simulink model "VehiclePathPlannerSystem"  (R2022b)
settings: Solver=VariableStepAuto  StartTime=0.0  StopTime=Tsim  RelTol=1e-3
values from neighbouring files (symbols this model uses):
  distToCenter = 0.5*egoWheelbase    [main.m]
  egoInitialPose = [1, 3, 0]    [main.m]
  egoLength = 4.7    [helperSLVisualizeParking.m]    (also in main.m = vdims.Length; parkingIneqConFcn.m = vdims.Length; parkingIneqConFcnJacobian.m = vdims.Length; parkingStateValidator.m)
  egoTargetPose = [-3.1, -3.15, pi/2]    [main.m]
  egoWheelbase = vdims.Wheelbase    [main.m]
  egoWidth = 1.8    [helperSLVisualizeParking.m]    (also in main.m = vdims.Width; parkingIneqConFcn.m = vdims.Width; parkingIneqConFcnJacobian.m = vdims.Width; parkingStateValidator.m)
  hp = 35    [main.m]    (also in parkingCostFcn.m = data.PredictionHorizon; parkingCostJacobian.m = data.PredictionHorizon; parkingIneqConFcn.m = data.PredictionHorizon; parkingIneqConFcnJacobian.m = data.PredictionHorizon)
  numObs = 8    [main.m]
  obsMat = [-9.3      , -1.75, 0,      egoLength,     egoWidth ;            -obsLength, -1.75, 0,      egoLength,     egoWidth ;             11.35    ,  1.35, 0,  4 * obsLength, 0.5          ;            -1.3      , -2   , 0,  0.5          , 1 + obsLength;            -obsLength, -5.35, 0, 10.3          , 0.5          ;            -11.1     , -2   , 0,  0.5          , 1 + obsLength;            -17.55    ,  1.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    [main.m]
  safetyDistance = 0.1    [main.m]
  steer_range = [-pi/5, pi/5]    [main.m]
  Ts = 0.1    [main.m]
  v_range = [-3.5, 3.5]    [main.m]
undefined symbols (not defined in the file or in its folder): blkObsMat, Column, D, egoParas, numParas, repmat, Row, vector
libraries: mpclib x1

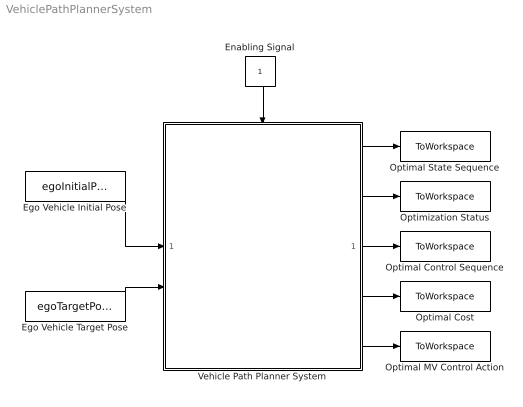
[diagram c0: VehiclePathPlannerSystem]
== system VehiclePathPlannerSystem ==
  Ego Vehicle Initial Pose : Constant  Value=egoInitialPose  VectorParams1D=off
  Ego Vehicle Target Pose : Constant  Value=egoTargetPose  VectorParams1D=off
  Enabling Signal : Constant
  Optimal Control Sequence : ToWorkspace  VariableName=mv_seq  SampleTime=-1
  Optimal Cost : ToWorkspace  VariableName=cost  SampleTime=-1
  Optimal MV Control Action : ToWorkspace  VariableName=mv_opti  SampleTime=-1
  Optimal State Sequence : ToWorkspace  VariableName=x_seq  SampleTime=-1
  Optimization Status : ToWorkspace  VariableName=exitflag  SampleTime=-1
  Vehicle Path Planner System : Subsystem  AncestorBlock=mpclib/Automated Driving/Vehicle Path Planner System  TreatAsAtomicUnit=on  mask(Vehicle Path Planner (VPP) system){egoLength=egoLength, egoWidth=egoWidth, wheelbase=egoWheelbase, dist2Center=distToCenter, numObs=numObs, obsMat=obsMat, obs_ext=off, minDist=safetyDistance, Ts=Ts, pPlanning=hp, v_range=v_range, v_ext=off, steer_range=steer_range, steer_ext=off, suboptimal=off, maxiter=200, output_exitflag=on}
      mask prompts: egoLength "MPC:adasblocks:promptCPPLength"; egoWidth "MPC:adasblocks:promptCPPWidth"; wheelbase "MPC:adasblocks:promptCPPWheelbase"; dist2Center "MPC:adasblocks:promptCPPCenterToRear"; numObs "MPC:adasblocks:promptCPPNumObs"; obsMat "MPC:adasblocks:promptCPPObsList"; obs_ext "MPC:adasblocks:promptCPPUseExternalSource"; minDist "MPC:adasblocks:promptCPPMinDist"; Ts "MPC:adasblocks:promptCPPSampleTime"; pPlanning "MPC:adasblocks:promptCPPSteps"; v_range "MPC:adasblocks:promptCPPVelRange"; v_ext "MPC:adasblocks:promptCPPUseExternalSource"; steer_range "MPC:adasblocks:promptCPPSteerRange"; steer_ext "MPC:adasblocks:promptCPPUseExternalSource"; suboptimal "MPC:adasblocks:promptCPPUseSubOptimal"; maxiter "MPC:adasblocks:promptCPPMaxIter"; output_exitflag "MPC:adasblocks:promptCPPExitflag"
      mask help: MPC:adasblocks:vppMaskDescription
      mask init:
      | [nlobj,numParas,egoParas,blkDataType,blkObsDim,blkObsMat] = vppblock_MaskInitFcn(gcb,pPlanning,Ts,...
      |     wheelbase,egoLength,egoWidth,dist2Center,minDist,...
      |     obsMat,numObs,v_range,steer_range,maxiter);
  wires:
  Enabling Signal/1 -> Vehicle Path Planner System/Enable
  Ego Vehicle Target Pose/1 -> Vehicle Path Planner System/2(Ego Vehicle Target Pose)
  Ego Vehicle Initial Pose/1 -> Vehicle Path Planner System/1(Ego Vehicle Initial Pose)
  Vehicle Path Planner System/2(Exitflag) -> Optimization Status/1
  Vehicle Path Planner System/1(Optimal State Sequence) -> Optimal State Sequence/1
  Vehicle Path Planner System/3(Optimal Control Sequence) -> Optimal Control Sequence/1
  Vehicle Path Planner System/4(Optimal Cost) -> Optimal Cost/1
  Vehicle Path Planner System/5(Optimal MV Control Action) -> Optimal MV Control Action/1

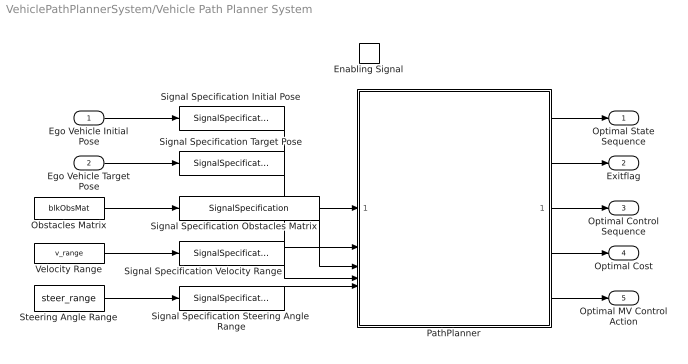
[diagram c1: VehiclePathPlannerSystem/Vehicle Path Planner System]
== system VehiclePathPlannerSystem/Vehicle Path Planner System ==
  Ego Vehicle Initial Pose : Inport
  Ego Vehicle Target Pose : Inport  Port=2
  Enabling Signal : EnablePort  StatesWhenEnabling=reset
  Obstacles Matrix : Constant  Value=blkObsMat  OutDataTypeStr=double
  PathPlanner : Subsystem
  Signal Specification Initial Pose : SignalSpecification  OutDataTypeStr=blkDataType  Dimensions=[1,3]
  Signal Specification Obstacles Matrix : SignalSpecification  OutDataTypeStr=blkDataType  Dimensions=blkObsDim
  Signal Specification Steering Angle Range : SignalSpecification  OutDataTypeStr=blkDataType  Dimensions=[1,2]
  Signal Specification Target Pose : SignalSpecification  OutDataTypeStr=blkDataType  Dimensions=[1,3]
  Signal Specification Velocity Range : SignalSpecification  OutDataTypeStr=blkDataType  Dimensions=[1,2]
  Steering Angle Range : Constant  Value=steer_range  OutDataTypeStr=double
  Velocity Range : Constant  Value=v_range  OutDataTypeStr=double
  Optimal State Sequence : Outport
  Exitflag : Outport  Port=2
  Optimal Control Sequence : Outport  Port=3
  Optimal Cost : Outport  Port=4
  Optimal MV Control Action : Outport  Port=5
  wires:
  Obstacles Matrix/1 -> Signal Specification Obstacles Matrix/1
  Steering Angle Range/1 -> Signal Specification Steering Angle Range/1
  Velocity Range/1 -> Signal Specification Velocity Range/1
  Signal Specification Steering Angle Range/1 -> PathPlanner/5(Steer Range)
  Signal Specification Velocity Range/1 -> PathPlanner/4(Velocity Range)
  Signal Specification Obstacles Matrix/1 -> PathPlanner/3(Obstacles Matrix)
  Signal Specification Target Pose/1 -> PathPlanner/2(Target Pose)
  Signal Specification Initial Pose/1 -> PathPlanner/1(Initial Pose)
  PathPlanner/1(Planned Path) -> Optimal State Sequence/1
  Ego Vehicle Target Pose/1 -> Signal Specification Target Pose/1
  Ego Vehicle Initial Pose/1 -> Signal Specification Initial Pose/1
  PathPlanner/2(Optimization status) -> Exitflag/1
  PathPlanner/3(Optimal Control Sequence) -> Optimal Control Sequence/1
  PathPlanner/4(Optimal Cost) -> Optimal Cost/1
  PathPlanner/5(Optimal MV Control Action) -> Optimal MV Control Action/1

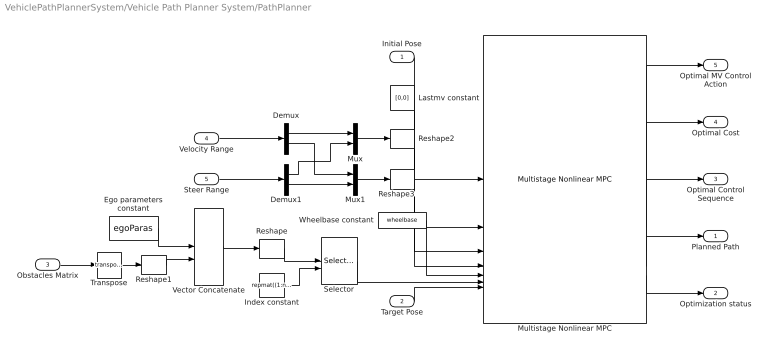
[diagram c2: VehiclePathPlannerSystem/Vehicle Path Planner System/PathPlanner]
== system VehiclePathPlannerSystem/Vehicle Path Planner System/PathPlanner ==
  Initial Pose : Inport
  Target Pose : Inport  Port=2
  Obstacles Matrix : Inport  Port=3
  Velocity Range : Inport  Port=4
  Steer Range : Inport  Port=5
  Demux : Demux  Outputs=[1,1]
  Demux1 : Demux  Outputs=[1,1]
  Ego parameters constant : Constant  Value=egoParas  VectorParams1D=off  OutDataTypeStr=blkDataType
  Index constant : Constant  Value=repmat((1:numParas)',pPlanning,1)  VectorParams1D=off  OutDataTypeStr=blkDataType
  Lastmv constant : Constant  Value=[0,0]  OutDataTypeStr=blkDataType
  Multistage Nonlinear MPC : mpclib/Multistage Nonlinear MPC  SCDEnableBlockLinearizationSpecification=on  nlmpcobj=nlobj  UseObjectTs=on  TsControl=2  UseMEX=off  md_enabled=off  stateparam_enabled=on  stageparam_enabled=on  cost_enabled=on  mvseq_enabled=on  stateseq_enabled=on  slack_enabled=off  status_enabled=on  mv_min=on  mv_max=on  mvrate_min=off  mvrate_max=off  state_min=off  state_max=off  terminal_state=on  nlp_initialize=off
  Mux : Mux  Inputs=2
  Mux1 : Mux  Inputs=2
  Reshape : Reshape  OutputDimensionality=Row vector (2-D)  OutputDimensions=[1,numParas]
  Reshape1 : Reshape  OutputDimensionality=Column vector (2-D)
  Reshape2 : Reshape  OutputDimensionality=Customize  OutputDimensions=[1,2]
  Reshape3 : Reshape  OutputDimensionality=Customize  OutputDimensions=[1,2]
  Selector : Selector  NumberOfDimensions=2  InputPortWidth=3  IndexOptions=Select all,Index vector (port)  Indices=[1 3],repmat([1:numParas]',pPlanning,1)  OutputSizes=1,1
  Transpose : Math  Operator=transpose
  Vector Concatenate : Concatenate
  Wheelbase constant : Constant  Value=wheelbase  OutDataTypeStr=blkDataType
  Planned Path : Outport
  Optimization status : Outport  Port=2
  Optimal Control Sequence : Outport  Port=3
  Optimal Cost : Outport  Port=4
  Optimal MV Control Action : Outport  Port=5
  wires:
  Selector/1 -> Multistage Nonlinear MPC/6
  Index constant/1 -> Selector/2
  Reshape3/1 -> Multistage Nonlinear MPC/4
  Reshape2/1 -> Multistage Nonlinear MPC/3
  Demux1/2 -> Mux1/2
  Demux1/1 -> Mux/2
  Steer Range/1 -> Demux1/1
  Demux/2 -> Mux1/1
  Mux1/1 -> Reshape3/1
  Demux/1 -> Mux/1
  Velocity Range/1 -> Demux/1
  Mux/1 -> Reshape2/1
  Reshape1/1 -> Vector Concatenate/2
  Transpose/1 -> Reshape1/1
  Ego parameters constant/1 -> Vector Concatenate/1
  Obstacles Matrix/1 -> Transpose/1
  Vector Concatenate/1 -> Reshape/1
  Initial Pose/1 -> Multistage Nonlinear MPC/1
  Multistage Nonlinear MPC/1 -> Optimal MV Control Action/1
  Lastmv constant/1 -> Multistage Nonlinear MPC/2
  Reshape/1 -> Selector/1
  Wheelbase constant/1 -> Multistage Nonlinear MPC/5
  Multistage Nonlinear MPC/5 -> Optimization status/1
  Multistage Nonlinear MPC/4 -> Planned Path/1
  Target Pose/1 -> Multistage Nonlinear MPC/7
  Multistage Nonlinear MPC/2 -> Optimal Cost/1
  Multistage Nonlinear MPC/3 -> Optimal Control Sequence/1
